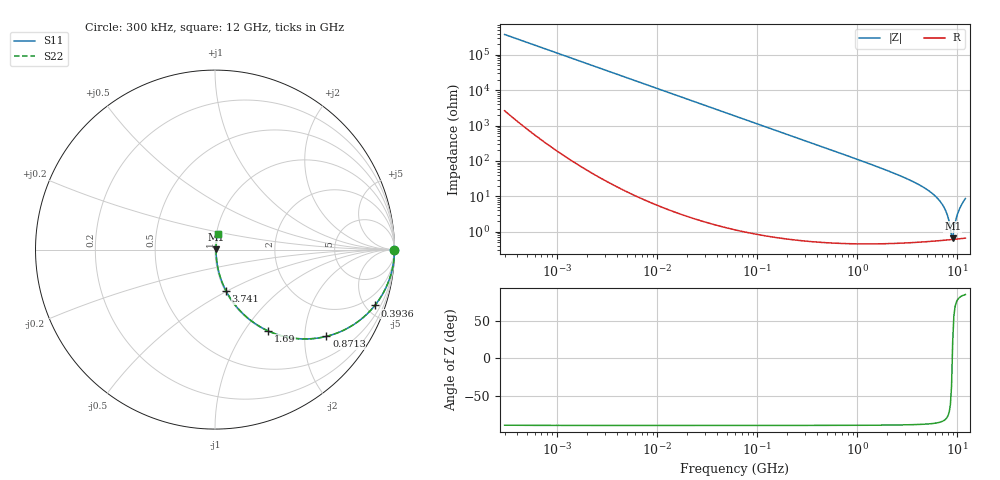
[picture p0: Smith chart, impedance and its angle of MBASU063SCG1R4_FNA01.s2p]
! MBASU063SCG1R4_FNA01  S-PARAMETER MODEL  ( General Type )
! Model Generated by TAIYO YUDEN Corporation (http://www.ty-top.com)
! Version 1.0
! TAIYO YUDEN Control No. 130801
! Copyright(c) 2013 TAIYO YUDEN CO.,LTD. All Rights Reserved.
! Product Description (link to TY-COMPAS)
! https://ds.yuden.co.jp/TYCOMPAS/or/detail?pn=MBASU063SCG1R4CFNA01&u=M
! Products Name : Multilayer Ceramic Capacitors
! Characteristics :
!  Capacitance : 1.4 pF , Rated Voltage : 50V , TCC : CG / C0G
!  Case Size : 0.6 x 0.3 / 0.024 x 0.012 [mm/inch] , Thickness : 0.3 / 0.012 [mm/inch]
!  (Conditions: Temperature = 25 degC , DC Bias Current/Voltage = 0A / 0V)
! External Node Assignments :
!  1  o---| |---o  2
! GND o---------o GND
! Frequency Range : 0.3MHz  -  12000MHz  [ 401 STEP ]
# MHz S RI R 50
! Freq[MHz].  S11 Real  S11 Imag  S21 Real  S21 Imag  S12 Real  S12 Imag  S22 Real  S22 Imag
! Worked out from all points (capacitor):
!   401 points, 300 kHz to 12 GHz, reference 50 ohm
!   read as one part in series: C = 1.41 pF near 316.3 kHz
!   lowest |Z| = 661 mohm at 8.967 GHz (marker M1)
!   series resonance near 8.88 GHz, so ESL is about 230 pH
!   S11 on the Smith chart (normalised r, x): 300 kHz: open; 393.6 MHz: 1.01, -5.72; 871.3 MHz: 1.01, -2.56; 1.69 GHz: 1.01, -1.29; 3.741 GHz: 1.01, -0.50; 12 GHz: 1.01, +0.17
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0.3  1 -0.000266  1.93e-06 0.000266  1.93e-06 0.000266  1 -0.000266
1.769972  1 -0.00157  4.12e-06 0.00157  4.12e-06 0.00157  1 -0.00157
10.44266  0.9999 -0.00926  9.03e-05 0.00926  9.03e-05 0.00926  0.9999 -0.00926
60  0.9971 -0.0531  0.00286 0.0531  0.00286 0.0531  0.9971 -0.0531
155.7172  0.9811 -0.1355  0.0189 0.1355  0.0189 0.1355  0.9811 -0.1355
353.9943  0.9096 -0.2859  0.0904 0.2859  0.0904 0.2859  0.9096 -0.2859
393.5654  0.8906 -0.3113  0.1094 0.3113  0.1094 0.3113  0.8906 -0.3113
871.3074  0.6212 -0.4833  0.3788 0.4833  0.3788 0.4833  0.6212 -0.4833
1689.663  0.294 -0.452  0.706 0.452  0.706 0.452  0.294 -0.452
2088.533  0.2086 -0.4018  0.7914 0.4018  0.7914 0.4018  0.2086 -0.4018
3740.715  0.0621 -0.2315  0.9379 0.2315  0.9379 0.2315  0.0621 -0.2315
5278.635  0.0238 -0.1343  0.9762 0.1343  0.9762 0.1343  0.0238 -0.1343
6699.894  0.0108 -0.0715  0.9892 0.0715  0.9892 0.0715  0.0108 -0.0715
7648.807  0.00722 -0.0377  0.9928 0.0377  0.9928 0.0377  0.00722 -0.0377
8064.993  0.00647 -0.0244  0.9935 0.0244  0.9935 0.0244  0.00647 -0.0244
8503.825  0.00608 -0.0111  0.9939 0.0111  0.9939 0.0111  0.00608 -0.0111
8732.115  0.00601 -0.00439  0.994 0.00439  0.994 0.00439  0.00601 -0.00439
8966.534  0.00605 0.00258  0.994 -0.00258  0.994 -0.00258  0.00605 0.00258
9207.246  0.00617 0.00923  0.9938 -0.00923  0.9938 -0.00923  0.00617 0.00923
9968.853  0.00711 0.0296  0.9929 -0.0296  0.9929 -0.0296  0.00711 0.0296
10511.28  0.00827 0.044  0.9917 -0.044  0.9917 -0.044  0.00827 0.044
12000  0.014 0.0853  0.986 -0.0853  0.986 -0.0853  0.014 0.0853
